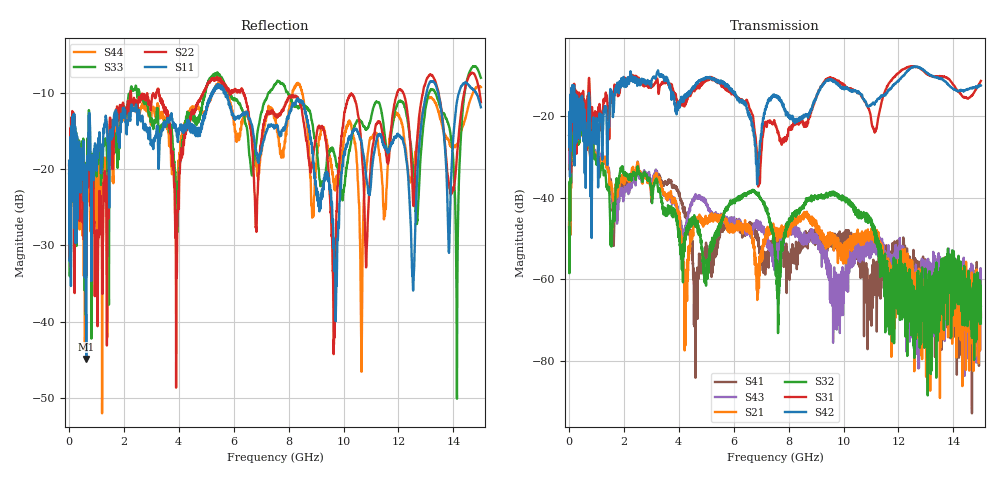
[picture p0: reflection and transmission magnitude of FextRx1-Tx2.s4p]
!  = SDD11
!  = SDD12
!  = SDC11
!  = SDC12
!  = SDD21
!  = SDD22
!  = SDC21
!  = SDC22
!  = SCD11
!  = SCD12
!  = SCC11
!  = SCC12
!  = SCD21
!  = SCD22
!  = SCC21
!  = SCC22
! FILE: N:\QM 2007\Prüfprotokolle\Highspeed\Konfektionierte Ltg\L45593-D106\D30\8216\0002\Fext\FextRx1-Tx2.s4p
# MHz S DB R 50.00
! FREQ  S11  S12  S13  S14
!  S21  S22  S23  S24
!  S31  S32  S33  S34
!  S41  S42  S43  S44
!  DB  ANG  DB  ANG  DB  ANG  DB  ANG
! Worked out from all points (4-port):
!   2999 points, 10 MHz to 15 GHz, reference 50 ohm
!   strongest paths, dB at 10 MHz, 3.755 GHz, 7.505 GHz, 11.26 GHz, 15 GHz:
!     S42: -24.8, -14.7, -15.2, -15.9, -12.7
!     S31: -24.7, -12.6, -22.1, -20.8, -11.5
!     S32: -47.3, -43.7, -54.5, -51.0, -70.7
!     S21: -46.8, -40.6, -47.9, -49.9, -69.0
!     S43: -45.0, -41.4, -54.0, -52.0, -69.3
!     S41: -46.3, -37.2, -49.6, -58.1, -66.4
!   lowest |S11| = -44.9 dB at 635 MHz (marker M1), VSWR 1.01, Z = 49.7 - j0.496 ohm
!   |S11| at or under -10 dB: start of sweep to 5.219 GHz; 5.701 GHz to 13.02 GHz (7.323 GHz wide, 78.2 % of centre); 13.44 GHz to 14.2 GHz (757.1 MHz wide, 5.48 % of centre)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
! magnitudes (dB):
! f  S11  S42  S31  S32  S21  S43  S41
! 10 MHz  -18.9  -24.8  -24.7  -47.3  -46.8  -45.0  -46.3
! 635 MHz  -44.9  -23.9  -27.3  -20.4  -20.7  -20.4  -20.7
! 4.615 GHz  -15.3  -12.6  -13.2  -47.1  -45.3  -39.1  -69.3
! 6.92 GHz  -18.6  -29.1  -36.8  -39.4  -62.1  -46.7  -51.8
! 9.655 GHz  -29.4  -11.5  -11.1  -39.2  -50.4  -59.8  -50.8
! 10.23 GHz  -16.1  -13.8  -13.4  -41.1  -50.6  -54.2  -51.0
! 15 GHz  -11.9  -12.7  -11.5  -70.7  -69.0  -69.3  -66.4
